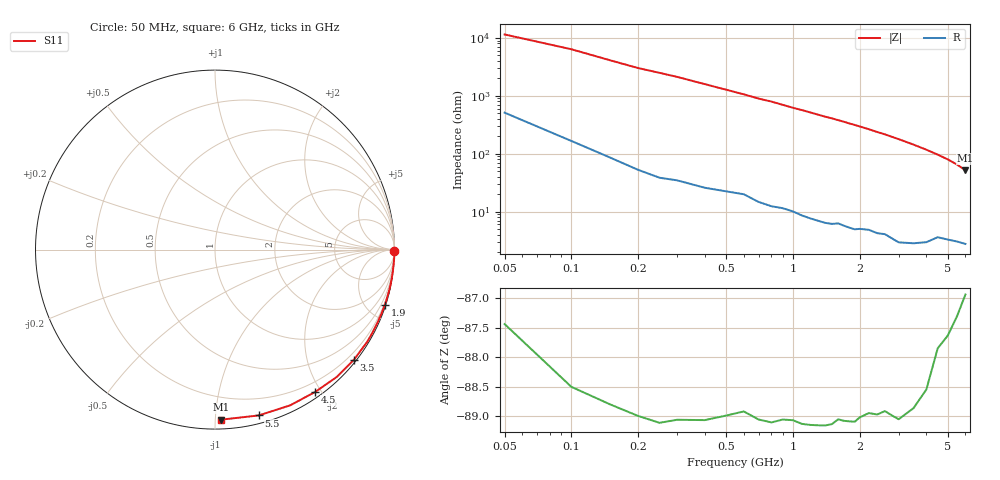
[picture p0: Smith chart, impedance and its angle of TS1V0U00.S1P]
! SIEMENS Small Signal Semiconductors
! BAT14-03W
! Si Schottky Diode in SOD323
! VR = 1 V
! S-Parameters:  November  1995
# GHz  S  MA  R  50
!  f  S11
! GHz  MAG  ANG
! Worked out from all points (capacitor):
!   34 points, 50 MHz to 6 GHz, reference 50 ohm
!   read as one part to ground: C = 259 fF near 50 MHz
!   lowest |Z| = 51.9 ohm at 6 GHz (marker M1)
!   S11 on the Smith chart (normalised r, x): 50 MHz: open; 1.9 GHz: 0.10, -6.28; 3.5 GHz: 0.06, -2.87; 4.5 GHz: 0.07, -1.93; 5.5 GHz: 0.06, -1.30; 6 GHz: 0.06, -1.04
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0.05  0.9996 -0.5
0.1  0.9996 -0.9
0.2  0.9994 -1.9
0.3  0.9992 -2.7
0.4  0.999 -3.6
0.6  0.9982 -5.4
0.7  0.9982 -6.4
0.8  0.998 -7.2
1  0.9974 -9.2
1.1  0.9973 -10.1
1.2  0.9971 -11.1
1.4  0.9967 -13.1
1.5  0.9964 -14.0
1.6  0.9957 -15.0
1.7  0.9956 -16.0
1.8  0.9953 -17.1
1.9  0.9951 -18.1
2.2  0.9933 -21.4
2.4  0.9928 -23.8
2.6  0.9917 -26.1
2.8  0.9916 -28.7
3  0.9915 -31.3
3.5  0.9878 -38.4
4  0.9819 -46.2
4.5  0.9698 -54.8
5  0.9635 -64.2
5.5  0.9556 -75.2
6  0.948 -87.9
